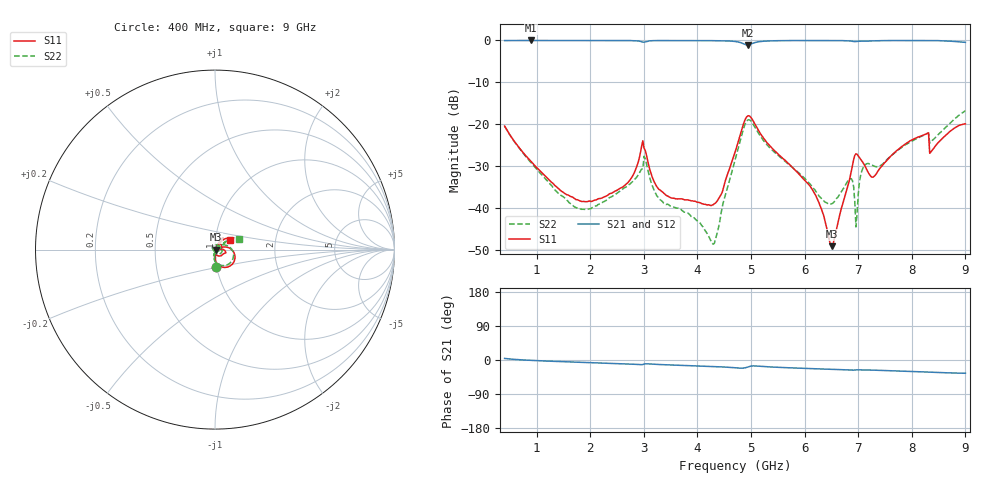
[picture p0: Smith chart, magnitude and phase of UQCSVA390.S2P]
!  Part Number  UQCSVA390  Mounting Orientation: Horizontal
!  Description: Ultra Low ESR Microwave capacitors
!  Application: Coupling, Bypass, Tuning, DC Block
!  Filters, Matching
# GHZ S DB R 50
! Freq  |S11|  S11 Ph  |S21|  S21 Ph  |S12|  S12 Ph  |S22|  S22 Ph
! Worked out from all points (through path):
!   401 points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, 400 MHz to 9 GHz, reference 50 ohm
!   highest |S21| = -0.01 dB at 895 MHz (marker M1); lowest = -1.1 dB at 4.937 GHz (marker M2)
!   group delay of S21, straight-line fit = 11.2 ps
!   lowest |S11| = -49.1 dB at 6.506 GHz (marker M3), VSWR 1.01, Z = 50.3 - j0.0762 ohm
!   |S11| at or under -10 dB: start of sweep to end of sweep
!   |S22| runs from -48.6 to -16.8 dB; largest |S21 - S12| = 0.0017
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0.4  -20.44 -85.3  -0.04 4.2  -0.05 4.1  -20.44 -85.5
0.895  -28.91 -86.8  -0.01 -1.0  -0.01 -1.1  -29.17 -93.6
1.841  -38.45 -48.8  -0.02 -6.2  -0.02 -6.2  -40.32 -152.9
2.658  -34.44 -8.5  -0.03 -10.2  -0.03 -10.2  -35.04 147.0
2.98  -23.94 -15.3  -0.41 -11.8  -0.40 -11.8  -30.66 33.5
3.045  -27.24 -56.7  -0.27 -10.0  -0.26 -10.1  -29.26 -48.4
3.281  -35.57 -76.7  -0.04 -11.9  -0.03 -11.9  -37.79 -102.5
3.969  -38.46 -56.6  -0.03 -15.5  -0.03 -15.5  -42.78 -137.3
4.292  -39.21 -22.7  -0.07 -17.3  -0.07 -17.3  -48.61 153.1
4.442  -36.73 4.8  -0.10 -18.2  -0.10 -18.2  -41.13 86.5
4.7  -26.70 17.9  -0.25 -20.5  -0.25 -20.5  -28.63 40.8
4.937  -18.02 -32.1  -1.07 -18.4  -1.08 -18.4  -19.00 -26.1
6.141  -35.57 -88.4  -0.02 -22.9  -0.02 -22.9  -34.92 -93.5
6.506  -49.11 -12.5  -0.03 -24.6  -0.04 -24.6  -38.98 -40.1
6.85  -32.51 69.2  -0.13 -26.6  -0.13 -26.7  -32.99 -15.1
6.958  -27.06 42.9  -0.27 -26.1  -0.27 -26.1  -44.52 -13.5
7.108  -29.58 17.6  -0.18 -26.4  -0.18 -26.4  -30.05 25.9
7.28  -32.62 37.7  -0.11 -26.7  -0.11 -26.7  -29.91 13.1
7.581  -27.95 59.7  -0.04 -28.2  -0.04 -28.2  -27.90 32.2
8.269  -22.32 57.3  -0.03 -31.7  -0.03 -31.7  -22.31 38.0
8.377  -26.26 53.1  -0.02 -32.2  -0.02 -32.2  -23.93 34.2
9  -19.92 31.2  -0.46 -34.9  -0.46 -34.9  -16.77 23.9
